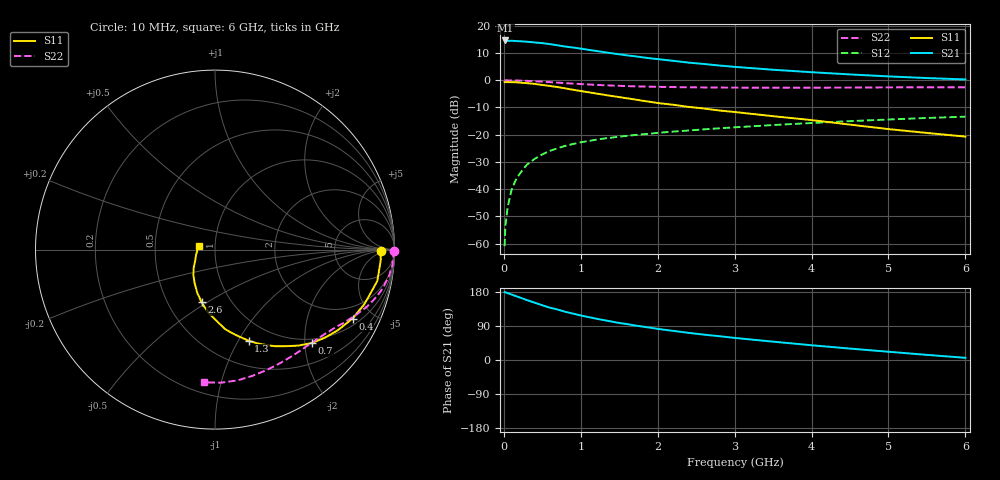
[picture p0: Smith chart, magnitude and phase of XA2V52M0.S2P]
! SIEMENS Discrete & RF Semiconductors
! BFY180
! Si NPN RF Bipolar Junction Transistor in MICRO-X
! VCE = 2.5 V  IC = 2 mA
! Common Emitter S-Parameters:  May  1997
# GHz  S  MA  R  50
!  f  S11  S21  S12  S22
! GHz  MAG  ANG  MAG  ANG  MAG  ANG  MAG  ANG
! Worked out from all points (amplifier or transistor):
!   36 points, 10 MHz to 6 GHz, reference 50 ohm
!   highest |S21| = 14.6 dB at 20 MHz (marker M1)
!   |S21| within 3 dB of that: start of sweep to 998.4 MHz
!   unconditionally stable (mu >= 1): 2.658 GHz to end of sweep
!   at 250 MHz: K = 0.12, MSG = 23.5 dB, |S12| = -32.7 dB
!   at 1.4 GHz: K = 0.71, MSG = 15.5 dB, |S12| = -21.1 dB
!   at 6 GHz: K = 1.07, MAG = 5.2 dB, |S12| = -13.4 dB
!   S11 on the Smith chart (normalised r, x): 10 MHz: 25, -2; 400 MHz: 1.31, -3.80; 700 MHz: 0.91, -2.16; 1.3 GHz: 0.77, -1.11; 2.6 GHz: 0.73, -0.47; 6 GHz: 0.83, +0.03
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0.01  0.9246 -0.4  5.303 179.2  0.0009 77.0  0.9955 -0.3
0.02  0.9222 -1.4  5.376 178.3  0.0021 89.9  0.9999 -0.6
0.05  0.9256 -3.5  5.269 176.5  0.0047 87.0  0.9953 -1.7
0.1  0.9217 -6.9  5.314 172.7  0.0097 85.8  0.9916 -3.4
0.15  0.921 -10.9  5.246 169.1  0.0143 84.0  0.9927 -5.1
0.3  0.8853 -20.2  5.101 158.1  0.0282 76.5  0.9738 -9.9
0.4  0.8574 -26.6  4.941 151.3  0.036 73.9  0.96 -12.9
0.5  0.8186 -33.3  4.8 144.4  0.0436 69.5  0.9414 -15.7
0.6  0.7854 -38.6  4.601 138.0  0.0507 66.5  0.9226 -18.2
0.7  0.7502 -43.9  4.378 133.1  0.0567 63.2  0.9041 -20.6
0.8  0.7078 -49.1  4.152 127.1  0.0625 60.8  0.8842 -22.7
0.9  0.6693 -53.5  3.99 122.4  0.0676 58.6  0.8676 -24.7
1.1  0.6026 -61.9  3.615 113.3  0.0766 54.3  0.8362 -28.2
1.3  0.5417 -69.7  3.283 105.3  0.0851 51.2  0.8097 -31.4
1.5  0.4907 -76.2  2.998 97.8  0.0922 48.7  0.7896 -34.3
1.7  0.4449 -83.0  2.762 91.3  0.0987 46.9  0.7734 -37.1
2.2  0.3551 -95.7  2.275 76.9  0.1141 42.6  0.7495 -43.8
2.6  0.3031 -104.3  1.99 67.0  0.1254 39.9  0.7381 -48.9
3.5  0.2189 -121.2  1.559 48.4  0.1505 33.8  0.7292 -60.3
4.5  0.1532 -140.5  1.279 30.1  0.1775 26.9  0.7337 -73.4
5.5  0.1078 -166.3  1.097 13.5  0.2031 19.3  0.7422 -87.5
6  0.0924 168.9  1.034 5.8  0.2145 15.1  0.7421 -94.6
